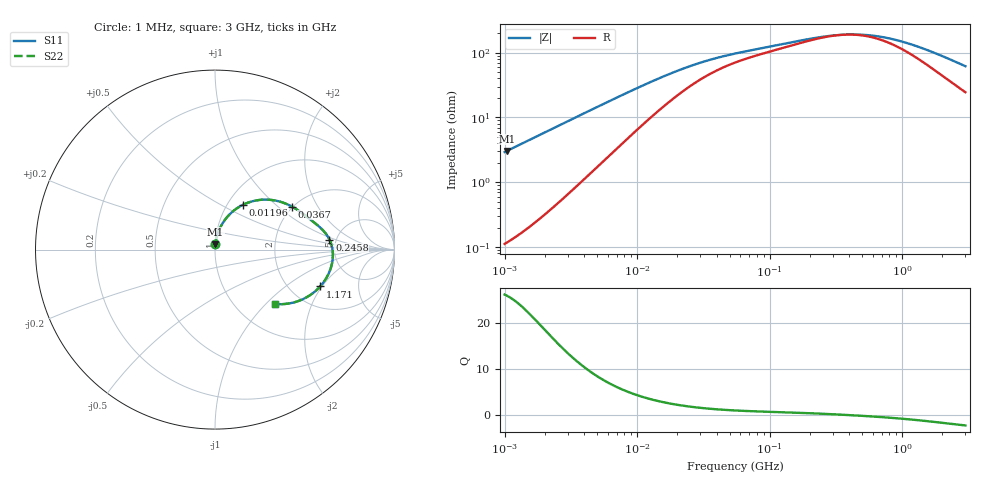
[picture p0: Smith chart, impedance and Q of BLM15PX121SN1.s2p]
! BLM15PX121SN1
# Hz S RI R 50
!Freq.(Hz) S11(Real) S11(Imag) S21(Real) S21(Imag) S12(Real) S12(Imag) S22(Real) S22(Imag)
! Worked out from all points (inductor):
!   401 points, 1 MHz to 3 GHz, reference 50 ohm
!   read as one part in series: L = 466 nH near 1.041 MHz
!   highest Q = 25.9 at 1.041 MHz (marker M1), where L = 466 nH
!   self-resonance near 365 MHz
!   S11 on the Smith chart (normalised r, x): 1 MHz: 1.00, +0.06; 11.96 MHz: 1.18, +0.65; 36.7 MHz: 1.98, +1.25; 245.8 MHz: 4.40, +0.83; 1.171 GHz: 2.88, -1.92; 3 GHz: 1.49, -1.14
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1000000  0.00197 0.0292  0.998 -0.0292  0.998 -0.0292  0.00197 0.0292
1040844  0.0021 0.0304  0.9979 -0.0304  0.9979 -0.0304  0.0021 0.0304
2097170  0.00712 0.0607  0.9929 -0.0607  0.9929 -0.0607  0.00712 0.0607
3823119  0.022 0.1076  0.978 -0.1076  0.978 -0.1076  0.022 0.1076
7110411  0.0685 0.1824  0.9315 -0.1824  0.9315 -0.1824  0.0685 0.1824
9223615  0.1059 0.2181  0.8941 -0.2181  0.8941 -0.2181  0.1059 0.2181
1.196486e7  0.1569 0.2502  0.8431 -0.2502  0.8431 -0.2502  0.1569 0.2502
1.461624e7  0.2046 0.2682  0.7954 -0.2682  0.7954 -0.2682  0.2046 0.2682
2.225279e7  0.3153 0.2765  0.6847 -0.2765  0.6847 -0.2765  0.3153 0.2765
3.670325e7  0.4286 0.2399  0.5714 -0.2399  0.5714 -0.2399  0.4286 0.2399
5.477226e7  0.4908 0.1992  0.5092 -0.1992  0.5092 -0.1992  0.4908 0.1992
2.094008e8  0.6269 0.0753  0.3731 -0.0753  0.3731 -0.0753  0.6269 0.0753
2.457655e8  0.6379 0.0555  0.3621 -0.0555  0.3621 -0.0555  0.6379 0.0555
3.385367e8  0.6528 0.0112  0.3472 -0.0112  0.3472 -0.0112  0.6528 0.0112
4.570858e8  0.6568 -0.0351  0.3432 0.0351  0.3432 0.0351  0.6568 -0.0351
6.049187e8  0.6508 -0.0823  0.3492 0.0823  0.3492 0.0823  0.6508 -0.0823
8.005644e8  0.6335 -0.1331  0.3665 0.1331  0.3665 0.1331  0.6335 -0.1331
1.171007e9  0.5859 -0.2053  0.4141 0.2053  0.4141 0.2053  0.5859 -0.2053
1.519029e9  0.5337 -0.2511  0.4663 0.2511  0.4663 0.2511  0.5337 -0.2511
1.970482e9  0.4652 -0.2863  0.5348 0.2863  0.5348 0.2863  0.4652 -0.2863
2.407135e9  0.4045 -0.3013  0.5955 0.3013  0.5955 0.3013  0.4045 -0.3013
3e9  0.3352 -0.303  0.6648 0.303  0.6648 0.303  0.3352 -0.303
